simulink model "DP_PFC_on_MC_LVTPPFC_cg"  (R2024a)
settings: Solver=FixedStepDiscrete  StartTime=0.0  StopTime=0.2  FixedStep=10e-6  RelTol=1e-3  EnableMultiTasking=on
model workspace (MAT data in the model file):
  Freq = 100
  Phas = 0
  SinFreq_1 = 250
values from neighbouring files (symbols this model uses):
  ADC = ADCType.Noise    [TotemPole_PFCData.m]
  Control = ControlType.Simple    [TotemPole_PFCData.m]
  Tsc_slow = 0.01    [TotemPole_PFCData.m]
undefined symbols (not defined in the file or in its folder): a, A0, A8, AD1, AD2, AD3, AD4, AD5, address, also, AN11, AN2, AN3, AN5, AN6, AppData, as, B0, B10, B11, B7, B8, below, bin2dec, bit, bits, BOR, C, C6, C7, C9, cause, characters, Code, Communicate, contains, counter, D, D4, Data, data, dead, default, Detailed, deviced, disasserted, DS70005539, dsPIC33AK128MC106, EC, ECIO, ensure, events, Family, faster, Floating, fulll, highest, HS, HS3, I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
libraries: MCHP_Blockset x16, simulink x4, dspswit3 x1
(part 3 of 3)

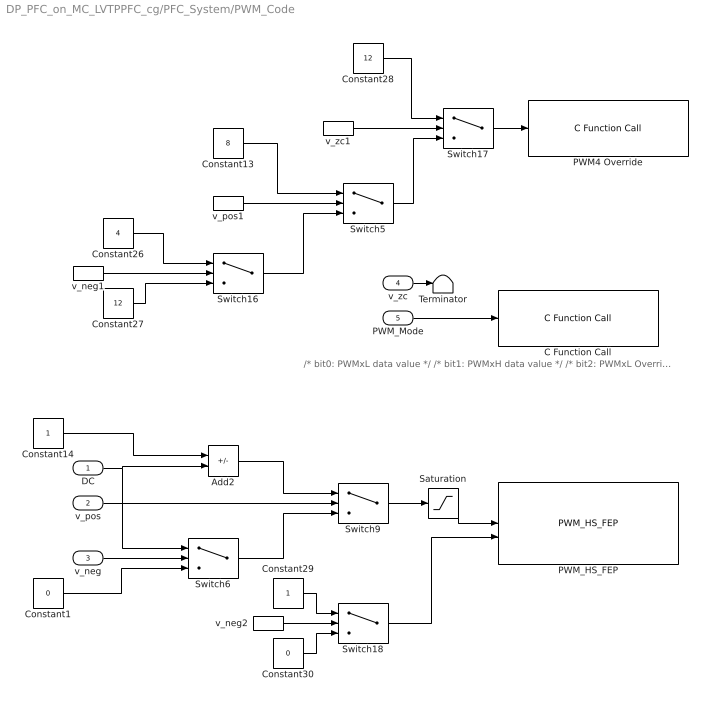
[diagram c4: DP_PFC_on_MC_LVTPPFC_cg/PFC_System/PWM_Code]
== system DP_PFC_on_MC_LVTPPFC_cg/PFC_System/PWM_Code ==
  note: /* bit0: PWMxL data value */ /* bit1: PWMxH data value */ /* bit2: PWMxL Override effective (1) */ /* bit3: PWMxH Override effective (1) */
  DC : Inport
  v_pos : Inport  Port=2
  v_neg : Inport  Port=3
  v_zc : Inport  Port=4
  PWM_Mode : Inport  Port=5
  Add2 : Sum  Inputs=+-
  C Function Call : MCHP_Blockset/User Functions/C Function Call  Priority=-5500  ParseFilesChkbx=on  ListFunctions1=Custom Function  Function1=void PWM1_Override(unsigned int OVER)  AddHeaderDeclaration=off  Function1Type=when block is updated (default)  Fct1BlockIn=OVER  FctReturnBlockOut=on  DataCollected="s.chksm={ '56741281'};s.File1={ '  void  PWM1_Override(unsigned int OVER)'};"  ORDERING=None  SampleTime=-1  S_INPUT=0  S_INPUT_Size=0  S_OUTPUT=0  S_OUTPUT_Size=0  S_ListCustomDatatype=0  MCHP_CRC=974059  MCHP_MASTERLINK=TotemPole_PFC_CodeGen/PFC_System/Control Variant /Microchip Master1  PinDigitalInput=[]  PinDigitalOutput=[]  PinAnalogInput=[]
  Constant1 : Constant  Value=0  OutDataTypeStr=single
  Constant13 : Constant  Value=8  OutDataTypeStr=uint16
  Constant14 : Constant  OutDataTypeStr=single
  Constant26 : Constant  Value=4  OutDataTypeStr=uint16
  Constant27 : Constant  Value=12  OutDataTypeStr=uint16
  Constant28 : Constant  Value=12  OutDataTypeStr=uint16
  Constant29 : Constant
  Constant30 : Constant  Value=0
  PWM4 Override : MCHP_Blockset/User Functions/C Function Call  Priority=-5500  ParseFilesChkbx=on  ListFunctions1=Custom Function  Function1=void PWM4_Override(unsigned int OVER)  AddHeaderDeclaration=off  Function1Type=when block is updated (default)  Fct1BlockIn=OVER  FctReturnBlockOut=on  DataCollected="s.chksm={ '113682597'};s.File1=reshape({ '  void  PWM1_Override(unsigned int OVER)','  void  PWM4_Override(unsigned int OVER)'},1,2);"  ORDERING=None  SampleTime=-1  S_INPUT=0  S_INPUT_Size=0  S_OUTPUT=0  S_OUTPUT_Size=0  S_ListCustomDatatype=0  MCHP_CRC=1025611  MCHP_MASTERLINK=TotemPole_PFC_CodeGen/PFC_System/Control Variant /Microchip Master1  PinDigitalInput=[]  PinDigitalOutput=[]  PinAnalogInput=[]
  PWM_HS_FEP : MCHP_Blockset/PWM IO/PWM_HS_FEP  Priority=-2000  PWMx_MODSEL=Center Aligned  PWMx_CLKSEL=Use divider circuit  PWM_ClockResolution_DIVSEL=Dynamic Options  PWM_ClockResolution_DIVSEL_TXT=auto  PWM_ClockResolution_FSCL=Dynamic Options  PWM_ClockResolution_FSCL_TXT="Resol: 0.05(us)  -  MaxPer: 0.00328(s)"  PWM_ClockResolution_NoScaling=Dynamic Options  PWM_ClockResolution_NoScaling_TXT="Resol: 0.005(us)  -  MaxPer: 0.000328(s)"  MaxPeriod_s=10e-6  InitPeriode_s=10e-6  InitDutyCycleP_s=0  InitDutyCycleS_s=10e-6  InitPhase_s=-1  evalin_ws=PWM1max=MCHP_Fun.Hex2num('408F400000000001');PWM4max=MCHP_Fun.Hex2num('408F400000000001');  SampleTime=-1  S_INPUT=[-1]  S_INPUT_Size=[3]  S_OUTPUT=[]  S_OUTPUT_Size=[]  S_ListCustomDatatype=S.S_ListCustomDatatype={};  MCHP_USER_INTERRUPTS=0  MCHP_PORT={PWMH1 }{PWMH1}32:4:D2;{PWMH4 }{PWMH4}32:4:C2;{PWML1}{PWML1}32:4:D3;{PWML4}{PWML4}32:4:C5;  MCHP_MASTERLINK=TotemPole_PFC_CodeGen/PFC_System/Control Variant /Microchip Master1  MCHP_CRC=4792858  PWMx_PMOD=Complementary  PWM1_HL=PWMxH & PWMxL output enabled  PWM1_swap=off  PWM1H_pol=off  PWM1L_pol=off  PWM2_HL=not used  PWM2_swap=off  PWM2H_pol=off  PWM2L_pol=off  PWM3_HL=not used  PWM3_swap=off  PWM3H_pol=off  PWM3L_pol=off  PWM4_HL=PWMxH & PWMxL output enabled  PWM4_swap=off  PWM4H_pol=off  PWM4L_pol=off  PWM5_HL=not used  PWM5_swap=off  PWM5H_pol=off  PWM5L_pol=off  PWM6_HL=not used  PWM6_swap=off  PWM6H_pol=off  PWM6L_pol=off  PWM7_HL=not used  PWM7_swap=off  PWM7H_pol=off  PWM7L_pol=off  PWM8_HL=not used  PWM8_swap=off  PWM8H_pol=off  PWM8L_pol=off  PWM9_HL=not used  PWM9_swap=off  PWM9H_pol=off  PWM9L_pol=off  PWM10_HL=not used  PWM10_swap=off  PWM10H_pol=off  PWM10L_pol=off  PWM11_HL=not used  PWM11_swap=off  PWM11H_pol=off  PWM11L_pol=off  PWM12_HL=not used  PWM12_swap=off  PWM12H_pol=off  PWM12L_pol=off  PWM1_ShowTrig=on  PWM1_Init_PGxTRIGABC_s=[0 -1 -1 ]  PWM1_ADTRxEN1=ADC Trigger 1  PWM1_ADTRxEN2=none  PWM1_ADTRxEN3=none  PWM2_ShowTrig=off  PWM2_Init_PGxTRIGABC_s=[-1 -1 -1]  PWM2_ADTRxEN1=none  PWM2_ADTRxEN2=none  PWM2_ADTRxEN3=none  PWM3_ShowTrig=off  PWM3_Init_PGxTRIGABC_s=[-1 -1 -1]  PWM3_ADTRxEN1=none  PWM3_ADTRxEN2=none  PWM3_ADTRxEN3=none  PWM4_ShowTrig=off  PWM4_Init_PGxTRIGABC_s=[-1 -1 -1]  PWM4_ADTRxEN1=none  PWM4_ADTRxEN2=none  PWM4_ADTRxEN3=none  PWM5_ShowTrig=off  PWM5_Init_PGxTRIGABC_s=[-1 -1 -1]  PWM5_ADTRxEN1=none  PWM5_ADTRxEN2=none  PWM5_ADTRxEN3=none  PWM6_ShowTrig=off  PWM6_Init_PGxTRIGABC_s=[-1 -1 -1]  PWM6_ADTRxEN1=none  PWM6_ADTRxEN2=none  PWM6_ADTRxEN3=none  PWM7_ShowTrig=off  PWM7_Init_PGxTRIGABC_s=[-1 -1 -1]  PWM7_ADTRxEN1=none  PWM7_ADTRxEN2=none  PWM7_ADTRxEN3=none  PWM8_ShowTrig=off  PWM8_Init_PGxTRIGABC_s=[-1 -1 -1]  PWM8_ADTRxEN1=none  PWM8_ADTRxEN2=none  PWM8_ADTRxEN3=none  BlockInput_VectorScalar=Independant Scalar  BlockInput_Period=Not a block input  BlockInput_DutyCycle=a Floating Point input within range [0 1]  BlockInput_PhaseShift=Not a block input  BlockInput_SEVTCMP=Not a block input  BlockInput_TRIGx=Not a block input  BlockInput_DeadTime=Not a block input  BlockOutput_FaultDisabled=off  BlockOutput_Fault=on  DTC=Positive dead time (ensure period of time with PWM_H and PWM_L disasserted)  FLTSRC1_DTCMP=Dynamic Options  FLTSRC1_DTCMP_TXT=<empty>  FLTSRC2_DTCMP=Dynamic Options  FLTSRC2_DTCMP_TXT=<empty>  FLTSRC3_DTCMP=Dynamic Options  FLTSRC3_DTCMP_TXT=<empty>  FLTSRC4_DTCMP=Dynamic Options  FLTSRC4_DTCMP_TXT=<empty>  FLTSRC5_DTCMP=Dynamic Options  FLTSRC5_DTCMP_TXT=<empty>  FLTSRC6_DTCMP=Dynamic Options  FLTSRC6_DTCMP_TXT=<empty>  FLTSRC7_DTCMP=Dynamic Options  FLTSRC7_DTCMP_TXT=<empty>  FLTSRC8_DTCMP=Dynamic Options  FLTSRC8_DTCMP_TXT=<empty>  FLTSRC9_DTCMP=Dynamic Options  FLTSRC9_DTCMP_TXT=<empty>  FLTSRC10_DTCMP=Dynamic Options  FLTSRC10_DTCMP_TXT=<empty>  FLTSRC11_DTCMP=Dynamic Options  FLTSRC11_DTCMP_TXT=<empty>  FLTSRC12_DTCMP=Dynamic Options  FLTSRC12_DTCMP_TXT=<empty>  DeadTime_s=150e-9  DeadTimeAlt_s=150e-9  DeadTimeComp_s=0  FLTMODx=Disabled  FLTSRCx=Dynamic Options  FLTSRCx_TXT=<empty>  FLTDATx=PWM H/L -> 11  CLMODx=Disabled  CLSRCx=Dynamic Options  CLSRCx_TXT=<empty>  CLDATx=PWM H/L -> 00  FLTLEBENx=off  CLLEBENx=off  LeadEdgeBlkPer_s=5e-7  PHRx=off  PHFx=off  PLRx=off  PLFx=off
  Saturation : Saturate  UpperLimit=1  LowerLimit=0
  Switch{5..6,9,16..18} (6 alike) : Switch  Criteria=u2 > Threshold
  Terminator : Terminator
  v_neg1 : InportShadow  Port=3
  v_neg2 : InportShadow  Port=3
  v_pos1 : InportShadow  Port=2
  v_zc1 : InportShadow  Port=4
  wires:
  PWM_Mode/1 -> C Function Call/1
  Switch6/1 -> Switch9/3
  DC/1 -> Switch6/1, Add2/2
  Add2/1 -> Switch9/1
  v_neg/1 -> Switch6/2
  Constant14/1 -> Add2/1
  Switch9/1 -> Saturation/1
  v_pos/1 -> Switch9/2
  Constant1/1 -> Switch6/3
  Saturation/1 -> PWM_HS_FEP/1
  v_zc/1 -> Terminator/1
  Constant27/1 -> Switch16/3
  Switch5/1 -> Switch17/3
  v_zc1/1 -> Switch17/2
  Switch16/1 -> Switch5/3
  Constant26/1 -> Switch16/1
  Constant13/1 -> Switch5/1
  v_neg1/1 -> Switch16/2
  Constant28/1 -> Switch17/1
  v_pos1/1 -> Switch5/2
  Switch17/1 -> PWM4 Override/1
  Constant29/1 -> Switch18/1
  v_neg2/1 -> Switch18/2
  Constant30/1 -> Switch18/3
  Switch18/1 -> PWM_HS_FEP/2

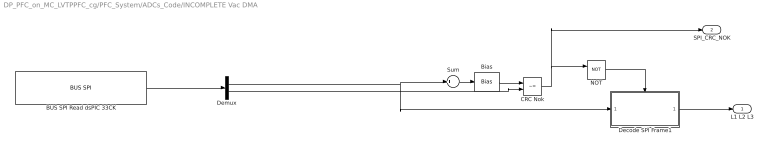
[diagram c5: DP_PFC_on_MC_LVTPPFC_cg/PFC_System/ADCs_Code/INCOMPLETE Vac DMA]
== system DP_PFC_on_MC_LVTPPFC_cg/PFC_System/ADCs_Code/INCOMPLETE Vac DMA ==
  BUS SPI Read dsPIC 33CK : MCHP_Blockset/BUS SPI/BUS SPI  SPIRef=1  DMA="[1  2  3]"  SPI_IntPriority=7  SPIsequence_txt="Initial-Configuration$     ---     $Set Port C8 / Pin[33] to 1$Set Port C8 / Pin[33] to 1$Set Port C8 / Pin[33] to 1$Set Port C8 / Pin[33] to 0$Read only (x4)  Read:{datas}"  SPIsequence_num=[BFF0000000000000 40A88E0000000000 0000000000000000 40E0000000000000 411E848000000000 411E848000000000]$4070000000000000$[4010000000000000 4044000000000000 3FF0000000000000]$[4010000000000000 4044000000000000 3FF0000000000000]$[4010000000000000 4044000000000000 3FF0000000000000]$[4010000000000000 4044000000000000 0000000000000000]$[4000000000000000 4010000000000000]  PIN_SDI_TXT=D4 / P53 / Pin[61]  PIN_SDO_TXT=C9 / P42 / Pin[34]  PIN_SCK_TXT=B11 / P28 / Pin[32]  PIN_SS_TXT=A0 / P1 / Pin[1]  S_INPUT="[5  5]"  S_OUTPUT=[5]  S_INPUT_Size="[2  2]"  S_OUTPUT_Size=[4]  BlockingMode=off  SampleTime=10e-6  MCHP_MASTERLINK=TotemPole_PFC_CodeGen/PFC_System/Control Variant /Microchip Master1  MCHP_PORT={SPI 1 input}{SDI1}12:0:P53;{SPI 1 Clock input}{SCK1_in}12:0:P28;{SPI 1 Digital output}{SPI1-DOU}12:1:C8;  ORDERING=0
  Bias : Bias  Bias=0x55
  CRC Nok : RelationalOperator  Operator=~=  OutDataTypeStr=boolean  RndMeth=Simplest
  Decode SPI Frame1 : Subsystem
  Demux : Demux  Outputs=[3 1]
  NOT : Logic  Operator=NOT  IconShape=distinctive  AllPortsSameDT=off  OutDataTypeStr=boolean
  Sum : Sum  Inputs=+
  L1 L2 L3 : Outport
  SPI_CRC_NOK : Outport  Port=2
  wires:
  Demux/1 -> Sum/1, Decode SPI Frame1/1(Frame)
  Demux/2 -> CRC Nok/2
  Bias/1 -> CRC Nok/1
  Sum/1 -> Bias/1
  NOT/1 -> Decode SPI Frame1/Enable
  Decode SPI Frame1/1(L1 L2 L3) -> L1 L2 L3/1
  CRC Nok/1 -> SPI_CRC_NOK/1, NOT/1
  BUS SPI Read dsPIC 33CK/1 -> Demux/1

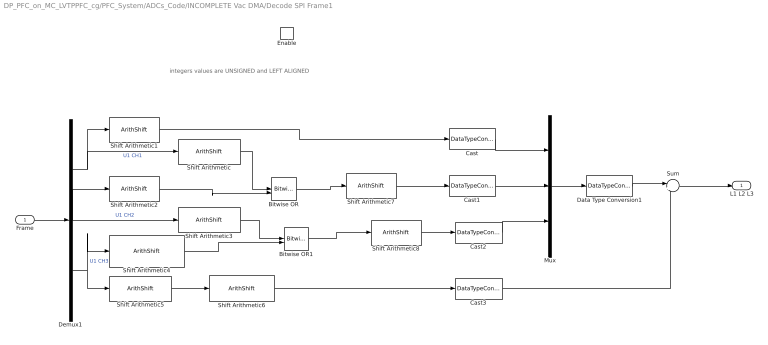
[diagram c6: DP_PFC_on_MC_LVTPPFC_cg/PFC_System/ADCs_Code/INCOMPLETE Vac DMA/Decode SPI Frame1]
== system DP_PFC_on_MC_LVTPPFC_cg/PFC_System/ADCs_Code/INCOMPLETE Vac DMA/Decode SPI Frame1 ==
  note: integers values are UNSIGNED and LEFT ALIGNED
  Frame : Inport
  Enable : EnablePort
  Bitwise OR : simulink/Logic and Bit Operations/Bitwise Operator  logicop=OR  UseBitMask=off  NumInputPorts=2  BitMask=bin2dec('11011001')  BitMaskRealWorld=Stored Integer
  Bitwise OR1 : simulink/Logic and Bit Operations/Bitwise Operator  logicop=OR  UseBitMask=off  NumInputPorts=2  BitMask=bin2dec('11011001')  BitMaskRealWorld=Stored Integer
  Cast : DataTypeConversion  OutDataTypeStr=uint16  ConvertRealWorld=Stored Integer (SI)
  Cast1 : DataTypeConversion  OutDataTypeStr=uint16  ConvertRealWorld=Stored Integer (SI)
  Cast2 : DataTypeConversion  OutDataTypeStr=uint16  ConvertRealWorld=Stored Integer (SI)
  Cast3 : DataTypeConversion  OutDataTypeStr=int16  ConvertRealWorld=Stored Integer (SI)
  Data Type Conversion1 : DataTypeConversion  OutDataTypeStr=int16
  Demux1 : Demux  Outputs=3
  Mux : Mux  Inputs=3
  Shift Arithmetic : ArithShift  BitShiftNumber=12  BitShiftDirection=Right
  Shift Arithmetic{1..2,6..8} (5 alike) : ArithShift  BitShiftNumber=4  BitShiftDirection=Left
  Shift Arithmetic3 : ArithShift  BitShiftNumber=8  BitShiftDirection=Right
  Shift Arithmetic4 : ArithShift  BitShiftNumber=8  BitShiftDirection=Left
  Shift Arithmetic5 : ArithShift  BitShiftNumber=4  BitShiftDirection=Right
  Sum : Sum  Inputs=|+-
  L1 L2 L3 : Outport
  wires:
  Shift Arithmetic5/1 -> Shift Arithmetic6/1
  Demux1/1 -> Shift Arithmetic1/1, Shift Arithmetic/1  "U1 CH1"
  Shift Arithmetic4/1 -> Bitwise OR1/2
  Demux1/3 -> Shift Arithmetic5/1, Shift Arithmetic4/1  "U1 CH3"
  Shift Arithmetic3/1 -> Bitwise OR1/1
  Demux1/2 -> Shift Arithmetic3/1, Shift Arithmetic2/1  "U1 CH2"
  Shift Arithmetic2/1 -> Bitwise OR/2
  Bitwise OR1/1 -> Shift Arithmetic8/1
  Shift Arithmetic6/1 -> Cast3/1
  Shift Arithmetic1/1 -> Cast/1
  Frame/1 -> Demux1/1
  Shift Arithmetic/1 -> Bitwise OR/1
  Bitwise OR/1 -> Shift Arithmetic7/1
  Cast/1 -> Mux/1
  Cast1/1 -> Mux/2
  Cast2/1 -> Mux/3
  Cast3/1 -> Sum/2
  Mux/1 -> Data Type Conversion1/1
  Shift Arithmetic7/1 -> Cast1/1
  Shift Arithmetic8/1 -> Cast2/1
  Sum/1 -> L1 L2 L3/1
  Data Type Conversion1/1 -> Sum/1
